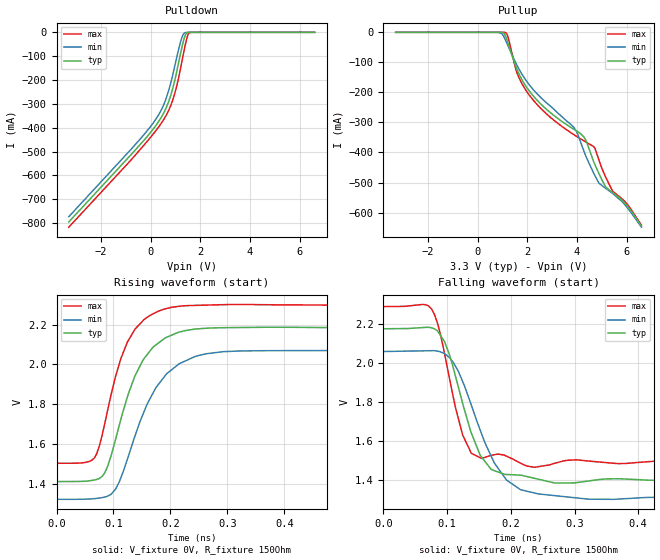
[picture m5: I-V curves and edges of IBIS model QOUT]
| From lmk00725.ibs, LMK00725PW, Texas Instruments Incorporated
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|   Model QOUT
[Model]   QOUT
Model_type   Output
Polarity   Non-Inverting
Vmeas = 1.65
Vref = 0
Cref = 15pF
Rref = 150
|   typ   min   max
|   (fast PVT)   (slow PVT)   (nom PVT)
C_comp   0.315p   0.300p   0.317p
|C_comp (Hi state)   0.315p   0.300p   0.317p
|C_comp (Low state)   0.358p   0.325p   0.360p
[Voltage Range]   3.3   3.1   3.5
[Temperature Range]   45   125   -40
[Pullup Reference]   3.3   3.1   3.5
[Pulldown Reference]   -0   0   0
[Power Clamp Reference]   3.3   3.1   3.5
[GND Clamp Reference]   0   0   0
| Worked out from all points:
|   slope of the pulldown table from 0 to 0.495 V, typ, clamps not added: 6.61 ohm
|   falling waveform, V_fixture 0V, R_fixture 150Ohm: 20-80 % time 42ps typ, 54.9ps min, 31.7ps max; typ from 2.18 V to 1.41 V
|   rising waveform, V_fixture 0V, R_fixture 150Ohm: 20-80 % time 54.1ps typ, 64.3ps min, 47.3ps max; typ from 1.41 V to 2.18 V
[Pulldown]
|   Voltage   I(typ)   I(min)   I(max)
-3.3V     -795mA     -773mA     -816.9mA
-260.7mV  -451mA     -427.3mA   -471.4mA
254.1mV   -383.6mA   -356.5mA   -405.7mA
531.3mV   -336.5mA   -301.6mA   -364.2mA
729.3mV   -288.1mA   -241.2mA   -325.7mA
917.4mV   -222.6mA   -164.7mA   -273.5mA
1.115V    -130.5mA   -74.41mA   -194.6mA
1.264V    -59.66mA   -19.11mA   -117.3mA
1.403V    -9.556mA   -957.4uA   -47.6mA
1.492V    -682.1uA   -81.19uA   -11.74mA
1.541V    -120.4uA   -20.08uA   -2.221mA
6.6V      3.471nA    3.392nA    3.552nA
[Pullup]
|   Voltage   I(typ)   I(min)   I(max)
-3.3V     0A         8.409pA    0A
848.1mV   -2.331uA   -203.3uA   -7.295nA
1.145V    -16.54mA   -29.93mA   -1.525mA
1.591V    -124.4mA   -110.4mA   -135.7mA
2.016V    -187.8mA   -167.7mA   -201.5mA
3.897V    -323.8mA   -318.7mA   -341.7mA
4.353V    -358.4mA   -410.4mA   -364.8mA
4.709V    -437.5mA   -474.7mA   -383.9mA
5.155V    -514.2mA   -518.9mA   -481.3mA
5.432V    -533.1mA   -535.8mA   -528mA
5.996V    -574.6mA   -580.3mA   -569.1mA
6.6V      -645mA     -648.6mA   -642.1mA
[Ramp]
R_load = 150
|   typ   min   max
dV/dt_r   0.460211/5.40957e-11   0.443898/6.42742e-11   0.473235/4.73097e-11
dV/dt_f   0.46012/4.20244e-11   0.443813/5.48766e-11   0.473292/3.16972e-11
[Falling Waveform]
V_fixture = 0V
V_fixture_min = 0V
V_fixture_max = 0V
R_fixture = 150Ohm
C_fixture = 0F
|   Time   V(typ)   V(min)   V(max)
0s        2.177V     2.06V      2.291V
74.84ps   2.183V     2.065V     2.282V
86.01ps   2.161V     2.062V     2.193V
103.7ps   2.044V     2.03V      1.923V
124.5ps   1.794V     1.906V     1.632V
152ps     1.528V     1.656V     1.515V
193.2ps   1.429V     1.401V     1.523V
237.3ps   1.41V      1.334V     1.466V
303.5ps   1.388V     1.309V     1.505V
2.85ns    1.41V      1.321V     1.502V
[Rising Waveform]
V_fixture = 0V
V_fixture_min = 0V
V_fixture_max = 0V
R_fixture = 150Ohm
C_fixture = 0F
|   Time   V(typ)   V(min)   V(max)
0s        1.41V      1.321V     1.502V
65.48ps   1.418V     1.324V     1.526V
80.13ps   1.436V     1.329V     1.645V
95.3ps    1.536V     1.345V     1.842V
124.5ps   1.837V     1.524V     2.113V
152ps     2.024V     1.751V     2.221V
174ps     2.097V     1.881V     2.262V
219.6ps   2.166V     2.009V     2.295V
362.1ps   2.187V     2.069V     2.301V
2.85ns    2.177V     2.061V     2.291V
